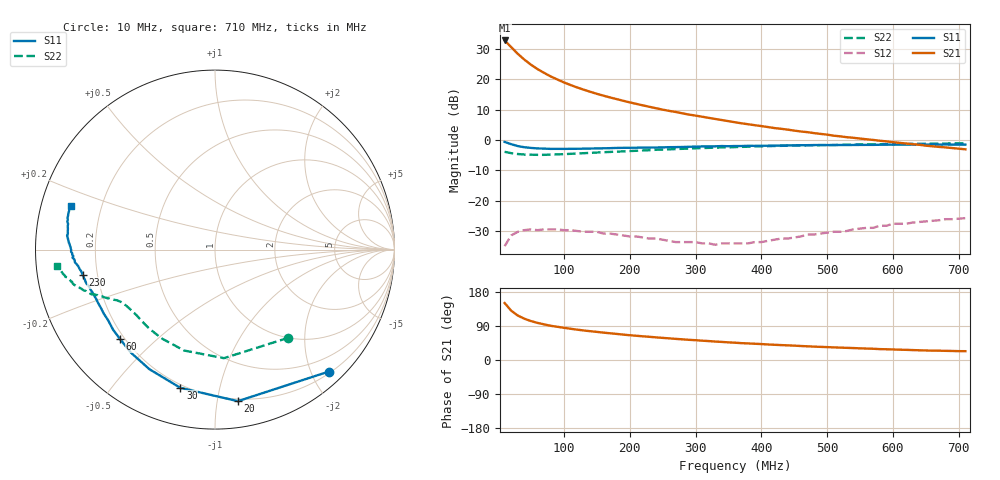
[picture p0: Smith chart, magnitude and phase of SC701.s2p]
!  POLYFET RF DEVICES
!  S PARAMETERS FOR
!  SC701
!  VDS=28, IDQ=200MA
! Date: Thu Jul 20 13:57:17 2000
# MHZ  S  MA  R  50.0000
! SCATTERING PARAMETERS :
! Freq=MHz Mag[s11] Ang[s11] Mag[s21] Ang[s21] Mag[s12] Ang[s12] Mag[s22] Ang[s22]
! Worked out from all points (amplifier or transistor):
!   71 points, 10 MHz to 710 MHz, reference 50 ohm
!   highest |S21| = 32.7 dB at 10 MHz (marker M1)
!   |S21| within 3 dB of that: start of sweep to 23.66 MHz
!   unconditionally stable (mu >= 1): 227.9 MHz to end of sweep
!   at 120 MHz: K = 0.43, MSG = 23.6 dB, |S12| = -29.9 dB
!   at 360 MHz: K = 1.74, MAG = 14.9 dB, |S12| = -34.0 dB
!   at 710 MHz: K = 1.27, MAG = 8.2 dB, |S12| = -25.7 dB
!   S11 on the Smith chart (normalised r, x): 10 MHz: 0.23, -2.28; 20 MHz: 0.18, -1.15; 30 MHz: 0.18, -0.76; 60 MHz: 0.18, -0.39; 230 MHz: 0.14, -0.09; 710 MHz: 0.09, +0.15
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10  0.929 -47.0  43.2 150.4  0.018 59.1  0.639 -50.3
20  0.854 -81.4  33.55 130.1  0.027 42.2  0.607 -85.3
30  0.794 -104.0  26.05 117.3  0.031 31.3  0.588 -107.0
40  0.76 -118.8  20.92 108.9  0.033 24.1  0.577 -120.6
50  0.741 -129.1  17.28 102.8  0.034 19.5  0.573 -129.4
60  0.727 -136.6  14.61 97.9  0.033 14.7  0.57 -135.7
70  0.722 -142.0  12.67 94.1  0.034 11.9  0.57 -140.2
80  0.714 -146.4  11.07 90.2  0.034 8.8  0.575 -143.4
90  0.715 -150.0  9.878 87.7  0.034 8.9  0.58 -146.0
100  0.714 -153.0  8.837 85.0  0.033 7.9  0.586 -147.9
110  0.716 -155.6  8.018 82.5  0.033 6.0  0.592 -149.5
130  0.72 -159.0  6.716 77.9  0.031 5.4  0.607 -151.8
150  0.728 -162.0  5.74 74.2  0.031 5.9  0.622 -153.1
170  0.734 -164.3  5.006 70.5  0.029 4.7  0.636 -154.3
200  0.744 -166.9  4.153 65.4  0.026 6.0  0.659 -155.7
230  0.751 -169.2  3.512 61.2  0.024 8.1  0.68 -157.4
250  0.756 -170.9  3.156 58.4  0.023 11.5  0.696 -158.2
290  0.773 -173.7  2.617 53.2  0.021 20.5  0.725 -159.9
360  0.796 -177.9  1.956 45.6  0.02 41.9  0.764 -162.6
480  0.825 175.2  1.298 35.3  0.028 69.7  0.816 -167.3
600  0.837 168.5  0.921 27.8  0.042 80.8  0.858 -170.9
710  0.839 163.0  0.702 23.3  0.052 85.0  0.884 -174.2
